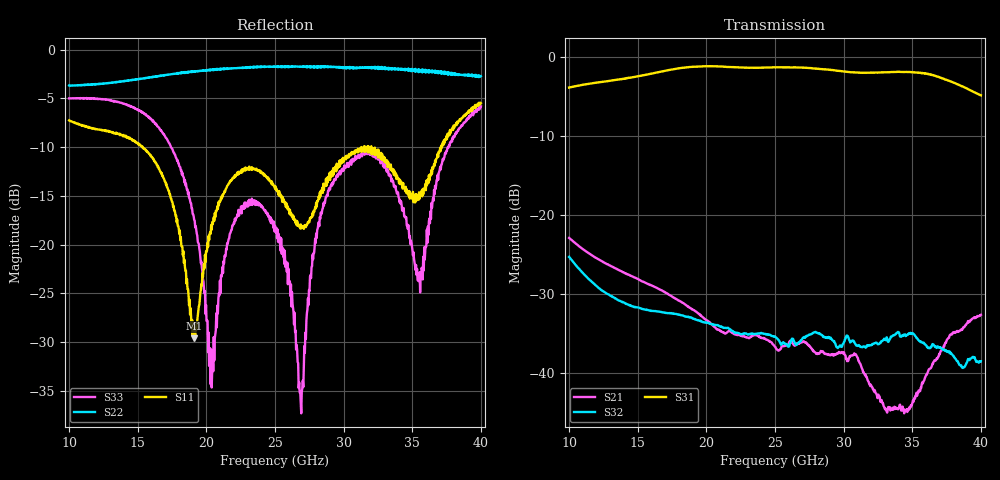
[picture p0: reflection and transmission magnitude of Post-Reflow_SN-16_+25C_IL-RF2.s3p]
!Agilent Technologies,N5245A,US49150155,A.09.90.19
!Agilent N5245A: A.09.90.19
!Date: Monday, November 12, 2018 23:21:45
!Correction: S11(Full 3 Port(1,2,3))
!S12(Full 3 Port(1,2,3))
!S13(Full 3 Port(1,2,3))
!S21(Full 3 Port(1,2,3))
!S22(Full 3 Port(1,2,3))
!S23(Full 3 Port(1,2,3))
!S31(Full 3 Port(1,2,3))
!S32(Full 3 Port(1,2,3))
!S33(Full 3 Port(1,2,3))
!S3P File: Measurements: <S11,S12,S13>,
!<S21,S22,S23>,
!<S31,S32,S33>:
# Hz S  dB  R 50
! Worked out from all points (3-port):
!   801 points, 10 GHz to 40 GHz, reference 50 ohm
!   strongest paths, dB at 10 GHz, 17.5 GHz, 25 GHz, 32.5 GHz, 40 GHz:
!     S31: -3.9, -1.6, -1.3, -2.0, -4.9
!     S32: -25.3, -32.5, -35.4, -36.4, -38.5
!     S21: -22.9, -30.3, -36.7, -42.9, -32.7
!   lowest |S11| = -29.6 dB at 19.11 GHz (marker M1), VSWR 1.07, Z = 46.9 - j0.979 ohm
!   |S11| at or under -10 dB: 15.37 GHz to 31.3 GHz (15.93 GHz wide, 68.3 % of centre); 31.3 GHz to 31.48 GHz (179.1 MHz wide, 0.571 % of centre); 32.02 GHz to 37.1 GHz (5.086 GHz wide, 14.7 % of centre)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
1e10  -7.26 8.1  -22.91 81.7  -3.89 -159.6
      -22.93 81.8  -3.68 60.5  -25.34 14.4
      -3.87 -159.3  -25.33 14.6  -5.01 -105.7
1.51375e10  -9.80 -144.2  -28.24 -11.2  -2.43 89.1
            -28.27 -10.9  -3.00 -42.5  -31.83 -76.3
            -2.40 89.5  -31.78 -75.8  -6.24 159.4
1.91125e10  -29.58 -161.7  -32.04 -84.0  -1.25 -0.8
            -32.08 -84.0  -2.22 -107.7  -33.23 -160.7
            -1.23 -0.3  -33.19 -160.2  -17.45 83.1
2.035e10  -17.99 -111.7  -33.83 -103.6  -1.19 -29.6
          -33.84 -103.4  -2.07 -125.9  -33.87 171.6
          -1.17 -29.2  -33.85 172.2  -30.78 130.2
2.21875e10  -12.87 -142.0  -35.22 -123.7  -1.32 -71.4
            -35.19 -123.5  -1.91 -149.6  -34.97 130.2
            -1.30 -70.8  -34.94 130.8  -17.26 177.1
2.5e10  -14.26 176.4  -36.71 -166.5  -1.33 -133.8
        -36.71 -166.6  -1.75 176.4  -35.44 64.0
        -1.31 -133.2  -35.43 64.5  -18.06 109.8
2.69125e10  -18.33 -176.1  -36.08 168.6  -1.36 -177.8
            -36.17 169.3  -1.76 154.0  -35.89 29.7
            -1.34 -177.0  -35.92 29.7  -37.29 -19.6
3.0775e10  -10.44 -179.0  -37.79 97.4  -1.99 93.7
           -37.54 97.9  -1.85 107.1  -36.16 -68.6
           -1.95 94.7  -36.13 -68.3  -11.19 167.6
3.49e10  -15.05 148.8  -44.23 81.7  -1.95 -4.9
         -44.13 83.5  -2.00 51.7  -35.06 -165.0
         -1.92 -4.0  -34.98 -165.0  -19.59 29.7
4e10  -5.50 117.6  -32.61 -7.8  -4.87 -137.7
      -32.67 -6.9  -2.73 -31.0  -38.65 -32.1
      -4.85 -136.6  -38.53 -32.1  -5.82 128.4
